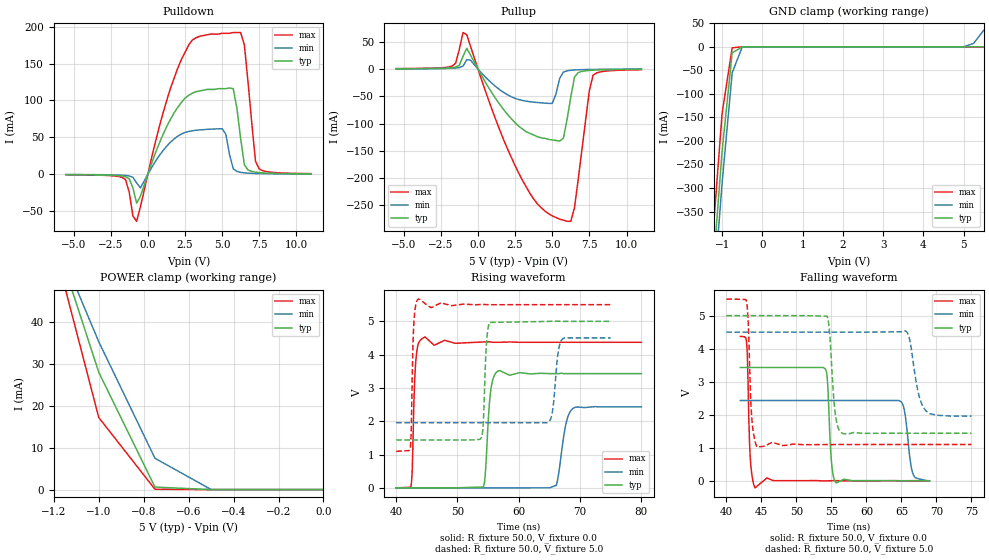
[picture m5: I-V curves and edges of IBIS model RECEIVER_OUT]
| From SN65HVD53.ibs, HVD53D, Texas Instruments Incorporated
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[Model]   RECEIVER_OUT
Model_type   3-state
| Signals   R
Vmeas = 2.2V   |Reference voltage for timing measurements
Cref = 15pF   |Timing specification test load capacitance value
Vref = 0   |Timing specification test load voltage; GND
| variable   typ   min   max
C_comp   25pF   20pF   30pF
|   typ   min   max
[Temperature Range]   25.0   -40   85
[Voltage range]   5.0V   4.5V   5.5V
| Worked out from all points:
|   slope of the pulldown table from 0 to 0.75 V, typ, clamps not added: 18.3 ohm
|   slope of the pullup table from 0 to 0.75 V, typ, clamps not added: 21.1 ohm
|   GND clamp passes 1 mA (typ) near -0.52 V on its own axis
|   POWER clamp passes 1 mA (typ) near -0.75 V on its own axis
|   rising waveform, R_fixture 50.0, V_fixture 0.0: 20-80 % time 683ps typ, 1.18ns min, 422ps max; typ from 0 V to 3.43 V
|   falling waveform, R_fixture 50.0, V_fixture 0.0: 20-80 % time 455ps typ, 788ps min, 333ps max; typ from 3.43 V to -0.001 V
|   rising waveform, R_fixture 50.0, V_fixture 5.0: 20-80 % time 457ps typ, 749ps min, 311ps max; typ from 1.44 V to 5 V
|   falling waveform, R_fixture 50.0, V_fixture 5.0: 20-80 % time 666ps typ, 1.24ns min, 447ps max; typ from 5 V to 1.44 V
[Pulldown]
|   Voltage   I(typ)   I(min)   I(max)
-5.5V     -420uA     -260uA     -560uA
-1.5V     -3.32mA    -1.54mA    -7.13mA
-750mV    -39.1mA    -11.6mA    -63.6mA
-500mV    -29.8mA    -18.4mA    -44.2mA
1.25V     63.7mA     37.6mA     98.5mA
2.75V     107mA      58.1mA     175mA
5V        116mA      61.8mA     191mA
5.75V     116mA      7.56mA     192mA
6.5V      12.8mA     2mA        175mA
7.25V     2.97mA     1.15mA     17.6mA
7.5V      2.39mA     1.01mA     7.26mA
11V       641uA      367uA      950uA
[Pullup]
|   Voltage   I(typ)   I(min)   I(max)
| Note that the[Pullup]voltage table is referenced to Vcc
| and is calculated using Vtable=Vcc - Vmeasured.
-5.5V     388uA      251uA      620uA
-1.75V    2.29mA     1.22mA     5.08mA
-1V       23.4mA     5.37mA     66.6mA
-750mV    37.7mA     17mA       62.6mA
3V        -110mA     -57.7mA    -204mA
5V        -130mA     -63.2mA    -269mA
5.75V     -127mA     -5.86mA    -277mA
6V        -92.7mA    -3.45mA    -279mA
6.5V      -14.7mA    -1.91mA    -254mA
7.5V      -2.71mA    -990uA     -39.3mA
7.75V     -2.27mA    -890uA     -11.4mA
11V       -190uA     -90uA      -1.5mA
[GND_clamp]
|   Voltage   I(typ)   I(min)   I(max)
| Outputs in High Impedance (off)
-5.5V     -5.07A     -5.05A     -5.12A
-1.25V    -500mA     -565mA     -423mA
-1V       -221mA     -289mA     -141mA
-750mV    -12.7mA    -55mA      -2.02mA
-500mV    -8.18uA    -416uA     -41.3uA
5V        65.5pA     16.7uA     61.8pA
5.25V     77.3pA     7.48mA     69.1pA
5.5V      47nA       35.3mA     74.6pA
[POWER_clamp]
|   Voltage  I(typ)   I(min)   I(max)
| Note that the [POWER_clamp] voltage table is referenced to Vcc
| and is calculated using Vtable = Vcc - Vmeasured.
| Outputs in Tri-state.
-5.5V     830mA      648mA      1.05A
-1.25V    69.2mA     67.2mA     68.8mA
-1V       28mA       35.3mA     17.2mA
-750mV    606uA      7.48mA     88.4uA
-500mV    47nA       16.7uA     12.1nA
0V        65.5pA     144pA      74.6pA
[Ramp]
|   typ   min   max
dV/dt_r   2.14V/569ns   1.53V/1170ps   2.64V/311ps
dV/dt_f   2.14V/561ps   1.53V/1240ps   2.64V/333ps
R_load = 50
[Rising Waveform]
R_fixture = 50.0
V_fixture = 0.0
C_fixture = 0p
L_fixture = 0n
|   V(typ)   V(min)   V(max)
40ns      3.04uV     3uV        293uV
42.4ns    2.06uV     4.91uV     46.5mV
43.2ns    14.1uV     4.33uV     3.81V
44.2ns    36.2uV     3.07uV     4.48V
54.2ns    25.8mV     13.1uV     4.38V
55.4ns    2.89V      16.1uV     4.38V
56.6ns    3.51V      19.5uV     4.37V
66.1ns    3.43V      75.6mV     4.37V
68.8ns    3.43V      2.38V      4.37V
80ns      3.43V      2.43V      4.37V
[Falling Waveform]
R_fixture = 50.0
V_fixture = 0.0
C_fixture = 0p
L_fixture = 0n
|   V(typ)   V(min)   V(max)
42ns      3.43V      2.43V      4.37V
42.9ns    3.43V      2.43V      4.18V
43.4ns    3.43V      2.43V      744mV
44.1ns    3.43V      2.43V      -216mV
54ns      3.41V      2.43V      -4.55mV
55ns      593mV      2.43V      498uV
55.6ns    -49.7mV    2.43V      2.48mV
64.6ns    -98.1uV    2.43V      -31.8uV
66.7ns    1.11mV     184mV      -22uV
69ns      -525uV     -9.82mV    18.2uV
[Rising Waveform]
R_fixture = 50.0
V_fixture = 5.0
V_fixture_min = 4.5
V_fixture_max = 5.5
C_fixture = 0p
L_fixture = 0n
|   V(typ)   V(min)  V(max)
40ns      1.438V     1.957V     1.097V
42.3ns    1.438V     1.957V     1.202V
42.8ns    1.438V     1.957V     4.656V
43.5ns    1.438V     1.957V     5.651V
53.8ns    1.481V     1.957V     5.505V
54.2ns    1.918V     1.957V     5.506V
55.2ns    4.967V     1.957V     5.498V
64.8ns    4.997V     1.965V     5.5V
67ns      5V         4.442V     5.5V
75ns      5V         4.5V       5.5V
[Falling Waveform]
R_fixture = 50.0
V_fixture = 5.0
V_fixture_min = 4.5
V_fixture_max = 5.5
C_fixture = 0p
L_fixture = 0n
|   V(typ)   V(min)  V(max)
40ns      5V         4.5V       5.5V
42.9ns    5V         4.5V       5.415V
43.6ns    5V         4.5V       1.989V
44.4ns    5V         4.5V       1.017V
54.4ns    4.982V     4.5V       1.095V
55.5ns    2.119V     4.5V       1.096V
56.5ns    1.445V     4.5V       1.098V
65.6ns    1.439V     4.533V     1.097V
68.4ns    1.438V     2.141V     1.097V
75ns      1.438V     1.957V     1.097V
